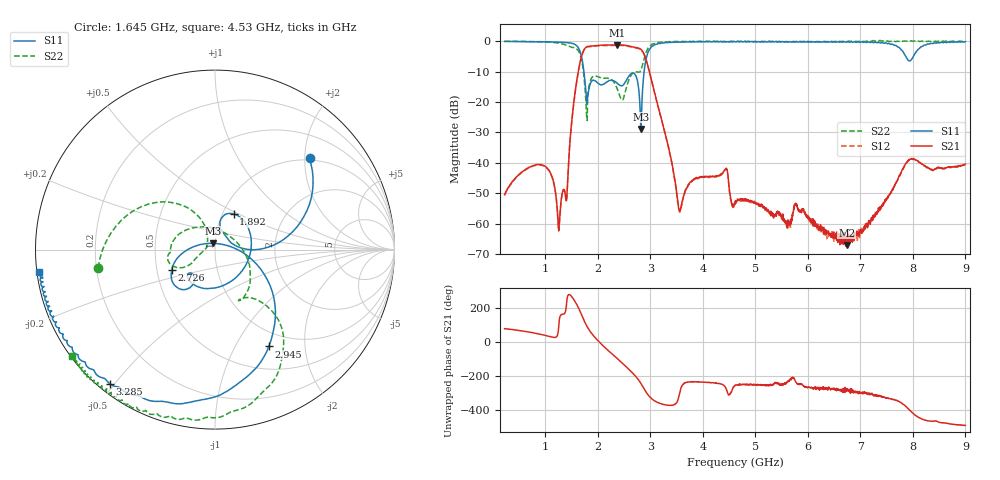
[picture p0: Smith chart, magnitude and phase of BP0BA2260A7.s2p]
!Agilent Technologies,E8358A,US41080443,A.07.50.56
!Agilent E8358A: A.07.50.56
!Date: Thursday, November 09, 2017 08:55:36
!Correction: S11(Full 2 Port(1,2))
!S21(Full 2 Port(1,2))
!S12(Full 2 Port(1,2))
!S22(Full 2 Port(1,2))
!S2P File: Measurements: S11, S21, S12, S22:
# Hz S  dB  R 50
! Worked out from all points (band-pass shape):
!   1601 points, 225 MHz to 9 GHz, reference 50 ohm
!   highest |S21| = -1.20 dB at 2.369 GHz (marker M1); lowest = -67.0 dB at 6.74 GHz (marker M2)
!   |S21| within 3 dB of the highest: 1.703 GHz to 2.88 GHz (1.176 GHz wide, 51.3 % of centre)
!   lowest |S11| = -28.9 dB at 2.819 GHz (marker M3), VSWR 1.07, Z = 49 + j3.43 ohm
!   |S11| at or under -10 dB: 1.735 GHz to 2.881 GHz (1.146 GHz wide, 49.7 % of centre)
!   |S22| runs from -26.1 to 0.3 dB; largest |S21 - S12| = 0.017
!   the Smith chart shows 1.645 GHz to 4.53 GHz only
!   S11 on the Smith chart (normalised r, x): 1.645 GHz: 0.96, +2.11; 1.892 GHz: 1.13, +0.47; 2.726 GHz: 0.60, -0.15; 2.945 GHz: 0.79, -1.38; 3.285 GHz: 0.03, -0.49; 4.53 GHz: 0.01, -0.06
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2.25e8  -0.08 172.2  -50.47 76.0  -50.57 77.2  0.01 168.5
9.489375e8  -0.19 143.0  -40.70 40.8  -40.88 40.9  -0.18 119.9
1.267031e9  -0.34 121.0  -60.24 127.8  -60.54 126.0  -0.66 64.2
1.524797e9  -0.80 84.0  -22.78 -104.1  -22.90 -104.3  -2.04 -74.0
1.645453e9  -2.70 44.1  -8.33 -170.3  -8.46 -170.4  -3.62 -171.2
1.689328e9  -5.10 22.9  -5.00 159.1  -5.11 159.4  -6.02 154.0
1.89225e9  -12.97 62.6  -1.58 44.6  -1.72 44.8  -11.86 -159.5
2.369391e9  -13.82 -137.9  -1.20 -98.6  -1.37 -98.4  -15.61 132.1
2.725875e9  -11.45 -154.4  -2.07 154.6  -2.21 154.6  -10.03 -64.5
2.819109e9  -28.86 104.3  -2.67 115.7  -2.81 115.9  -9.58 -53.8
2.94525e9  -4.19 -60.9  -7.60 52.7  -7.76 52.8  -2.68 -60.1
3.153656e9  -0.75 -113.6  -21.74 1.3  -21.90 1.6  -0.43 -95.3
3.285281e9  -0.44 -128.0  -30.51 -10.9  -30.67 -10.4  -0.22 -106.6
3.5595e9  -0.28 -145.2  -55.82 56.8  -56.27 60.4  -0.03 -120.7
4.530234e9  -0.12 -172.8  -51.80 59.4  -51.80 59.0  -0.03 -143.3
4.6125e9  -0.18 -175.0  -53.61 102.7  -53.21 98.5  0.03 -145.7
6.076828e9  -0.27 150.8  -59.70 87.0  -59.04 92.5  -0.17 179.5
6.740438e9  -0.25 134.5  -67.03 84.3  -66.36 67.5  -0.08 163.5
7.541156e9  -0.69 99.5  -50.78 26.3  -50.69 27.3  -0.09 147.8
7.85925e9  -4.82 18.5  -40.43 -17.7  -40.58 -18.4  0.02 142.4
8.018297e9  -4.68 -108.7  -38.73 -64.5  -38.82 -64.3  0.06 141.7
9e9  -0.13 147.7  -40.36 -131.8  -40.57 -130.9  -0.06 133.5
